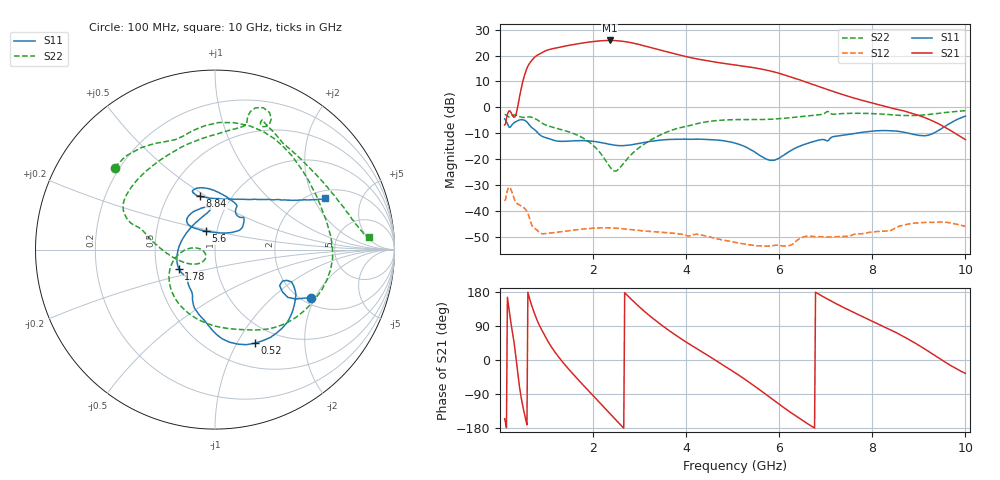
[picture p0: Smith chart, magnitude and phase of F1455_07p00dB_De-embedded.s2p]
! Integrated Device Technology
! Corporate Headquarters
! 6024 Silver Creek Valley Road
! San Jose, CA 95138  USA
! Phone:  1-408-284-8200
! Toll Free:  1-800-223-1366
! Webpage:  http://www.idt.com/
! Timing and RF Division
! 515 Groton Road, Suite 102
! Westford, MA 01886-6024
! Device:  F1455
! Description: 6-bit 0.5 dB Transmit Variable Gain Amplifier
! Frequency:  1400.0 -  2300.00 MHz
! Package:  6x6 mm Thin QFN Plastic Package: 28 pin
! State:  14
! Atten State:  7.0 dB
! Voltage:  +5.00 Volts
! Current:  217.704 mA
! Data:  The device was measured on a the F1455 evaluation board which has
!  individual transmission lines to the RF pins.  Data was collected
!  using a calibrated network analyzer.  The evaluation board was
!  de-embedded using a TRL calibration technique.
!  The reference plane is the edge of the package pin.
!  Pin  1 = CSb
!  Pin  2 = DATA
!  Pin  3 = CLK
!  Pin  4 = RSET
!  Pin  5 = GND
!  Pin  6 = RFIN  = Port 1
!  Pin  7 = GND
!  Pin  8 = NC
!  Pin  9 = NC
!  Pin 10 = NC
!  Pin 11 = NC
!  Pin 12 = NC
!  Pin 13 = NC
!  Pin 14 = /STBY
!  Pin 15 = GND
!  Pin 16 = RFOUT  = Port 2
!  Pin 17 = GND
!  Pin 18 = NC
!  Pin 19 = NC
!  Pin 20 = NC
!  Pin 21 = GND
!  Pin 22 = NC
!  Pin 23 = GND
!  Pin 24 = NC
!  Pin 25 = NC
!  Pin 26 = NC
!  Pin 27 = GND
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# GHz S dB R 50
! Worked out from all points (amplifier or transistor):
!   496 points, 100 MHz to 10 GHz, reference 50 ohm
!   highest |S21| = 25.8 dB at 2.36 GHz (marker M1)
!   |S21| within 3 dB of that: 1.177 GHz to 3.298 GHz (2.121 GHz wide, 94.8 % of centre)
!   unconditionally stable (mu >= 1): start of sweep to end of sweep
!   at 1.74 GHz: K = 5.76, MAG = 25.3 dB, |S12| = -47.1 dB
!   at 5.06 GHz: K = 19.50, MAG = 18.3 dB, |S12| = -52.1 dB
!   at 10 GHz: K = 57.64, MAG = -3.9 dB, |S12| = -45.9 dB
!   S11 on the Smith chart (normalised r, x): 100 MHz: 2.21, -1.86; 520 MHz: 0.77, -1.19; 1.78 GHz: 0.65, -0.15; 5.6 GHz: 0.88, +0.18; 8.84 GHz: 0.72, +0.47; 10 GHz: 2.35, +2.47
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0.1  -4.47 -26.9  -6.81 -155.1  -36.07 43.4  -2.83 140.8
0.38  -5.17 -38.3  0.07 -33.8  -37.27 -110.0  -3.26 56.0
0.52  -4.94 -67.1  11.92 -138.8  -38.86 -155.3  -3.91 23.6
0.7  -8.03 -98.9  18.48 137.3  -45.96 151.5  -3.92 -20.3
0.82  -10.00 -113.0  20.30 98.5  -47.80 136.2  -5.02 -48.5
0.96  -11.59 -120.3  21.66 65.0  -48.77 123.1  -6.64 -72.9
1.14  -12.65 -130.7  22.67 28.2  -48.39 100.3  -7.72 -97.7
1.34  -13.12 -136.6  23.45 -4.3  -47.93 77.8  -8.70 -121.4
1.76  -12.83 -151.2  24.78 -62.6  -47.00 42.0  -11.59 -159.3
1.78  -12.86 -152.2  24.84 -65.2  -46.98 40.6  -11.79 -160.9
2.08  -13.30 -169.2  25.56 -104.2  -46.58 19.4  -16.04 179.4
2.36  -14.28 166.4  25.82 -141.0  -46.52 1.4  -22.91 -177.9
2.74  -14.65 125.4  25.21 170.2  -47.05 -20.1  -19.74 -136.3
3.06  -13.68 102.7  23.94 133.0  -47.63 -34.2  -14.68 -156.9
3.4  -12.73 96.1  22.32 98.8  -48.12 -47.0  -11.07 -177.6
4.1  -12.31 112.6  19.17 39.7  -49.43 -68.7  -6.94 163.6
5.06  -13.84 136.8  16.36 -34.2  -52.12 -103.8  -4.74 148.3
5.6  -18.73 116.9  14.83 -80.4  -53.44 -110.1  -4.70 127.0
6.7  -13.38 42.2  8.98 -175.1  -49.79 -141.7  -3.15 78.3
8.36  -8.99 109.2  -0.07 81.1  -47.69 165.2  -2.79 62.2
8.84  -10.24 105.5  -2.20 50.3  -44.85 147.7  -3.16 43.9
10  -3.40 24.9  -12.48 -35.3  -45.94 77.6  -1.29 4.5
